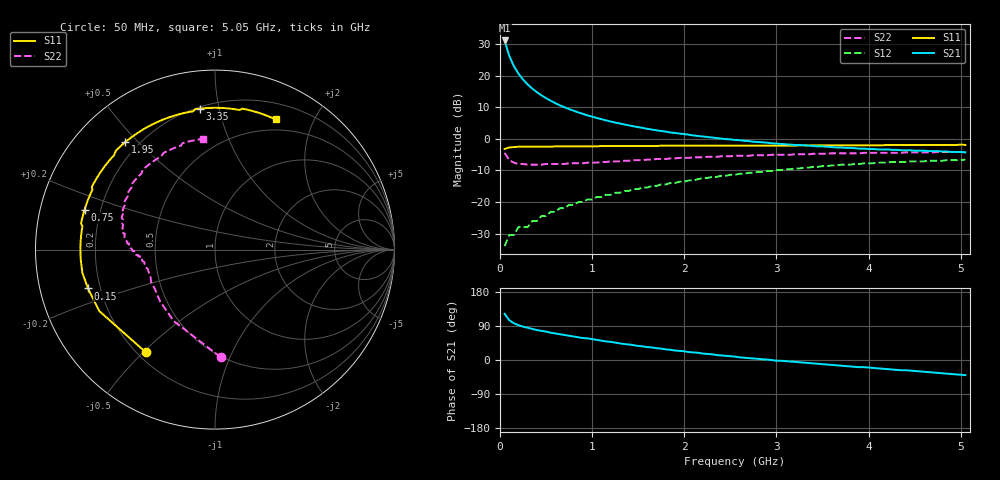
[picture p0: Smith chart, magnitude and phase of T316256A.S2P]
!AT-31625
!S-PARAMETERS at Vce=6.0 V  Ic=50 mA.  LAST UPDATED 08-05-96
# ghz s ma r 50
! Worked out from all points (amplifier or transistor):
!   101 points, 50 MHz to 5.05 GHz, reference 50 ohm
!   highest |S21| = 31.1 dB at 50 MHz (marker M1)
!   |S21| within 3 dB of that: start of sweep to 80.97 MHz
!   unconditionally stable (mu >= 1): 496.9 MHz to 507.2 MHz; 592.2 MHz to 609.5 MHz; 672.6 MHz to 1.336 GHz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
!   at 850 MHz: K = 1.01, MAG = 13.6 dB, |S12| = -20.0 dB
!   at 2.55 GHz: K = 0.93, MSG = 5.5 dB, |S12| = -11.4 dB
!   at 5.05 GHz: K = 0.95, MSG = 1.1 dB, |S12| = -6.6 dB
!   S11 on the Smith chart (normalised r, x): 50 MHz: 0.23, -0.51; 150 MHz: 0.15, -0.15; 750 MHz: 0.14, +0.15; 1.95 GHz: 0.15, +0.46; 3.35 GHz: 0.21, +0.88; 5.05 GHz: 0.37, +1.50
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0.05  0.69 -124.0  36.08 122.0  0.02 43.0  0.6 -87.0
0.1  0.73 -152.0  20.66 105.0  0.03 37.0  0.46 -120.0
0.15  0.74 -163.0  14.19 97.0  0.03 39.0  0.42 -137.0
0.2  0.75 -170.0  10.78 92.0  0.04 43.0  0.4 -147.0
0.25  0.75 -175.0  8.69 88.0  0.04 46.0  0.4 -153.0
0.3  0.75 -178.0  7.26 85.0  0.04 49.0  0.39 -157.0
0.35  0.75 179.0  6.25 82.0  0.05 52.0  0.39 -160.0
0.4  0.75 177.0  5.48 79.0  0.05 54.0  0.39 -162.0
0.45  0.75 174.0  4.88 77.0  0.06 55.0  0.39 -164.0
0.5  0.75 172.0  4.4 75.0  0.06 57.0  0.4 -166.0
0.6  0.76 169.0  3.68 70.0  0.07 59.0  0.4 -168.0
0.75  0.76 163.0  2.96 64.0  0.09 60.0  0.41 -171.0
0.9  0.76 159.0  2.48 58.0  0.1 60.0  0.41 -173.0
1.15  0.77 152.0  1.96 49.0  0.13 59.0  0.43 -176.0
1.35  0.77 146.0  1.69 42.0  0.15 57.0  0.45 -178.0
1.75  0.78 135.0  1.33 30.0  0.19 52.0  0.48 177.0
1.95  0.78 130.0  1.21 24.0  0.21 49.0  0.5 174.0
2.55  0.78 115.0  0.96 9.0  0.27 39.0  0.54 164.0
3.35  0.79 96.0  0.78 -8.0  0.35 25.0  0.57 148.0
3.4  0.79 95.0  0.77 -9.0  0.36 24.0  0.58 147.0
4.25  0.8 79.0  0.67 -25.0  0.43 5.0  0.6 123.0
5.05  0.8 65.0  0.61 -40.0  0.47 -12.0  0.62 96.0
